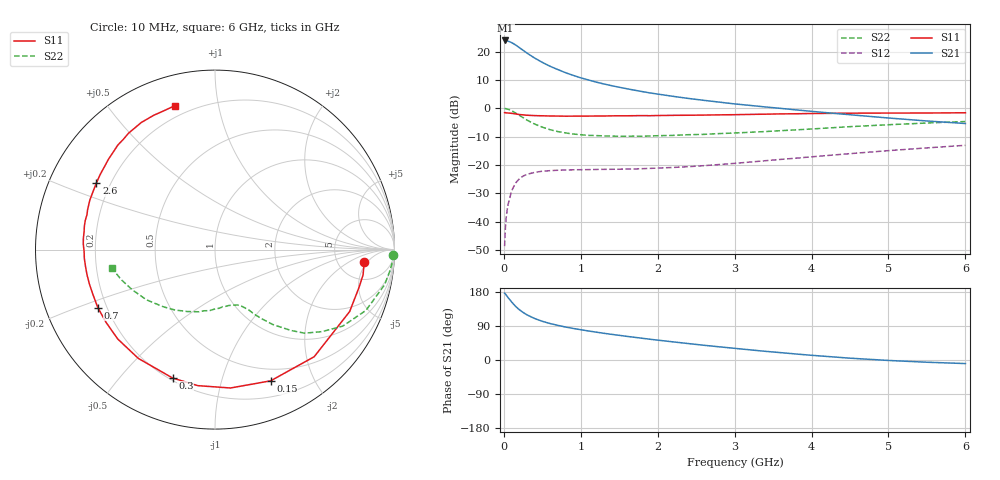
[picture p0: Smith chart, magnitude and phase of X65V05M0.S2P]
! SIEMENS Small Signal Semiconductors
! BFP193W
! Si NPN RF Bipolar Junction Transistor in SOT343
! VCE = 5 V  IC = 5 mA
! Common Emitter S-Parameters:  April 1994
# GHz  S  MA  R  50
!  f  S11  S21  S12  S22
! GHz  MAG  ANG  MAG  ANG  MAG  ANG  MAG  ANG
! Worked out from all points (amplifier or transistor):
!   40 points, 10 MHz to 6 GHz, reference 50 ohm
!   highest |S21| = 23.9 dB at 20 MHz (marker M1)
!   |S21| within 3 dB of that: start of sweep to 226.1 MHz
!   unconditionally stable (mu >= 1): 1.703 GHz to 4.342 GHz
!   at 200 MHz: K = 0.14, MSG = 23.2 dB, |S12| = -24.9 dB
!   at 1.5 GHz: K = 0.91, MSG = 14.5 dB, |S12| = -21.5 dB
!   at 6 GHz: K = 0.92, MSG = 3.8 dB, |S12| = -13.1 dB
!   lowest NFmin = 1.20 dB at 450 MHz
!   S11 on the Smith chart (normalised r, x): 10 MHz: 9, -4; 150 MHz: 0.37, -1.45; 300 MHz: 0.21, -0.70; 700 MHz: 0.17, -0.23; 2.6 GHz: 0.15, +0.26; 6 GHz: 0.14, +0.75
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0.01  0.8345 -4.8  15.64 176.3  0.0037 87.7  0.994 -1.6
0.02  0.8369 -9.7  15.68 174.4  0.0076 83.1  0.9879 -4.9
0.05  0.8258 -24.7  15.36 166.1  0.0188 76.9  0.9652 -11.7
0.1  0.8134 -47.2  14.38 153.4  0.0347 66.4  0.9069 -21.9
0.15  0.7942 -67.0  13.14 142.1  0.0476 56.7  0.8299 -30.9
0.2  0.7759 -83.6  11.75 132.9  0.0567 49.4  0.7509 -37.5
0.25  0.764 -97.2  10.53 125.6  0.0636 43.5  0.6827 -43.0
0.3  0.7535 -108.3  9.398 119.2  0.0683 38.4  0.6182 -46.8
0.4  0.7416 -125.2  7.682 109.5  0.074 32.0  0.5263 -52.4
0.5  0.736 -137.4  6.435 102.1  0.0776 28.0  0.4642 -56.0
0.6  0.7299 -146.3  5.503 96.3  0.0793 25.3  0.4191 -58.8
0.7  0.7285 -153.7  4.819 91.5  0.0807 23.8  0.3882 -60.6
0.9  0.7256 -164.8  3.804 83.3  0.0822 21.9  0.3515 -64.4
1.1  0.7276 -172.6  3.154 76.6  0.0828 21.5  0.3326 -67.9
1.3  0.7294 -179.3  2.681 70.5  0.0837 22.1  0.3254 -71.8
1.6  0.7361 172.2  2.207 62.3  0.0849 24.2  0.3212 -77.7
2.2  0.7499 158.5  1.622 47.8  0.0904 30.3  0.3323 -90.9
2.6  0.7579 150.6  1.379 38.9  0.0972 34.7  0.3461 -100.1
3.2  0.7785 139.6  1.122 26.8  0.1125 39.4  0.377 -113.7
4.5  0.8187 120.1  0.768 4.8  0.1583 41.6  0.4734 -143.8
5.5  0.8242 110.2  0.596 -5.9  0.2 38.2  0.5491 -162.3
6  0.8323 105.7  0.538 -9.4  0.2221 36.1  0.5831 -169.8
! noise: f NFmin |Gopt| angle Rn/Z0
0.45  1.2  0.26  102  0.14
0.9  1.25  0.38  145  0.12
1.8  2.05  0.56  -161  0.12
